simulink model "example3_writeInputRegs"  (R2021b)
settings: Solver=FixedStepDiscrete  StartTime=0.0  StopTime=inf  FixedStep=0.5  RelTol=1e-3
libraries: ModbusServerLib x3

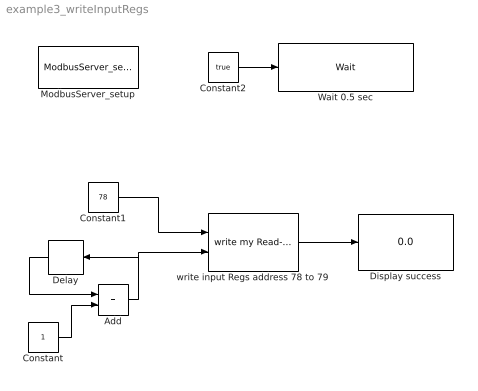
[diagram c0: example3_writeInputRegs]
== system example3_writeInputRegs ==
  Add : Sum
  Constant : Constant
  Constant1 : Constant  Value=78
  Constant2 : Constant  Value=true
  Delay : Delay  DelayLength=1
  Display success : Display
  ModbusServer_setup : ModbusServerLib/ModbusServer_setup  g1_cmbPortName="\"COM5\""  g2_cmbModbusType="\"Modbus RTU\""  g3_chkIgnoreServerID=off  g4_ObjectID=0  g5_ServerID=[1 2 3 4 5 ]  g30_TCPPort=502  g6_chkSupportDINCoil1to4=on  g7_HoldingRegsSeg1to4=[ 1,30 ; 35, 56]  g8_InputRegsSeg1to4=[1 44; 78 89]  g9_CoilSeg1to4=[1 44; 78 89]  g10_DiscreteSeg1to4=[1 44; 78 89]  g11_chkUseHoldingRegstoReplace1to4=off  g12_chkEnableWD1to4=off  g13_chkUseReadonlyRegs4WD1to4=off  g14_WDAddr1to4=1  g15_cmbWDType1to4=0  g16_WDPeriod1to4=20  g17_WDPreset1to4=20  g18_chkSupportDINCoil5=on  g19_HoldingRegsSeg5=[ 1,30 ; 35, 56]  g20_InputRegsSeg5=[1 44; 78 89]  g21_CoilSeg5=[1 44; 78 89]  g22_DiscreteSeg5=[1 44; 78 89]  g23_chkUseHoldingRegstoReplace5=off  g24_chkEnableWD5=off  g25_chkUseReadonlyRegs4WD5=off  g26_WDAddr5=1  g27_cmbWDType5=0  g28_WDPeriod5=20  g29_WDPreset5=20
  Wait 0.5 sec : ModbusServerLib/Wait  Waitms=500
  write input Regs address 78 to 79 : ModbusServerLib/write my Read-only Regs  g_ObjID=0  g_Endian=big-endian  g_DataType=uint32  g_DeviceNo=1
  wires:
  Add/1 -> Delay/1, write input Regs address 78 to 79/2
  Constant/1 -> Add/2
  Delay/1 -> Add/1
  Constant1/1 -> write input Regs address 78 to 79/1
  Constant2/1 -> Wait 0.5 sec/1
  write input Regs address 78 to 79/1 -> Display success/1
